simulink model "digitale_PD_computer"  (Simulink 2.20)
settings: Solver=VariableStepDiscrete  StartTime=0.0  StopTime=10.0  RelTol=1e-3  AbsTol=1e-6
libraries: Puma x1

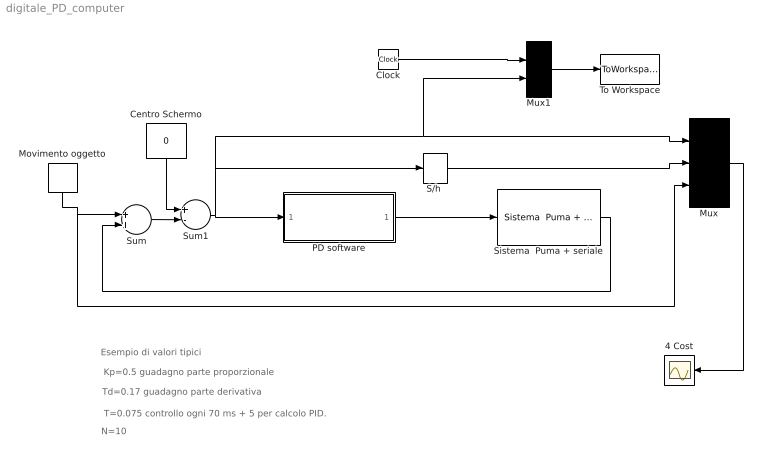
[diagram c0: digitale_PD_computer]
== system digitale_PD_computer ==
  note: Kp=0.5 guadagno parte proporzionale
  note: Td=0.17 guadagno parte derivativa
  note: T=0.075 controllo ogni 70 ms + 5 per calcolo PID.
  note: N=10
  note: Esempio di valori tipici
  4 Cost : Scope
  Centro Schermo : Constant  Orientation=down  Value=0
  Clock : Clock
  Movimento oggetto : DiscretePulseGenerator  Orientation=down  Amplitude=-47.5  Period=100  PulseWidth=100  PhaseDelay=1  SampleTime=.1
  Mux : Mux  Inputs=3
  Mux1 : Mux  Inputs=2
  PD software : Subsystem  mask(Simulazione PD implementato in maniera software){Kp=0.5, Td=0.17, T=0.070, N=10}
      mask prompts: Kp "Costante guadagno proporzionale"; Td "Costante di derivazione Td"; T "Sample Time T del PD"; N "Indice polo del derivatore [5..10]"
      mask init:
      | Kbeta=Td/(N*T+Td);
      | Kalfa=N*Kbeta;
      | 
      | U0=Kbeta;
      | E1=Kp*(1+Kalfa);
      | E0=-Kp*(Kbeta+Kalfa);
  "S/h " : ZeroOrderHold  SampleTime=.260
  Sistema  Puma + seriale : Puma/Sistema  Puma + seriale  Ts=.260
  Sum : Sum  Inputs=++
  Sum1 : Sum  Inputs=+-
  To Workspace : ToWorkspace  VariableName=sim  SampleTime=.01
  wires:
  Mux/1 -> 4 Cost/1
  Sum/1 -> Sum1/2
  Centro Schermo/1 -> Sum1/1
  Sum1/1 -> "S/h "/1, Mux/1, Mux1/2, PD software/1(In1)
  Movimento oggetto/1 -> Sum/1, Mux/3
  Clock/1 -> Mux1/1
  "S/h "/1 -> Mux/2
  Mux1/1 -> To Workspace/1
  Sistema  Puma + seriale/1 -> Sum/2
  PD software/1(Out1) -> Sistema  Puma + seriale/1

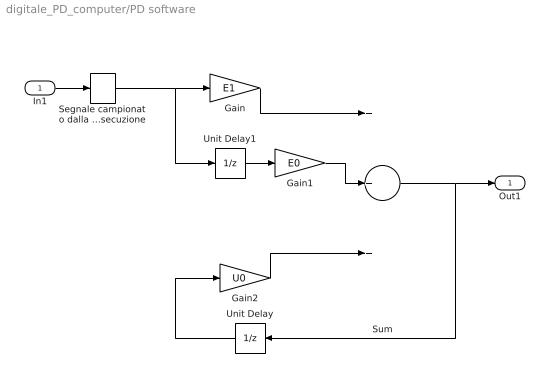
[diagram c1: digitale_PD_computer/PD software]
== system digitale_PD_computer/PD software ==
  In1 : Inport  Port=1  PortWidth=-1  SampleTime=-1
  Gain : Gain  Gain=E1
  Gain1 : Gain  Gain=E0
  Gain2 : Gain  Gain=U0
  Segnale campionato dalla procedura software al momento ciclo  di'esecuzione : ZeroOrderHold  SampleTime=T
  Sum : Sum  Inputs=+++
  Unit Delay : UnitDelay  Orientation=left  X0=0  SampleTime=T
  Unit Delay1 : UnitDelay  X0=0  SampleTime=T
  Out1 : Outport  Port=1
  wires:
  Gain1/1 -> Sum/2
  Unit Delay/1 -> Gain2/1
  Gain2/1 -> Sum/3
  Gain/1 -> Sum/1
  Unit Delay1/1 -> Gain1/1
  Sum/1 -> Out1/1, Unit Delay/1
  In1/1 -> Segnale campionato dalla procedura software al momento ciclo  di'esecuzione/1
  Segnale campionato dalla procedura software al momento ciclo  di'esecuzione/1 -> Gain/1, Unit Delay1/1
